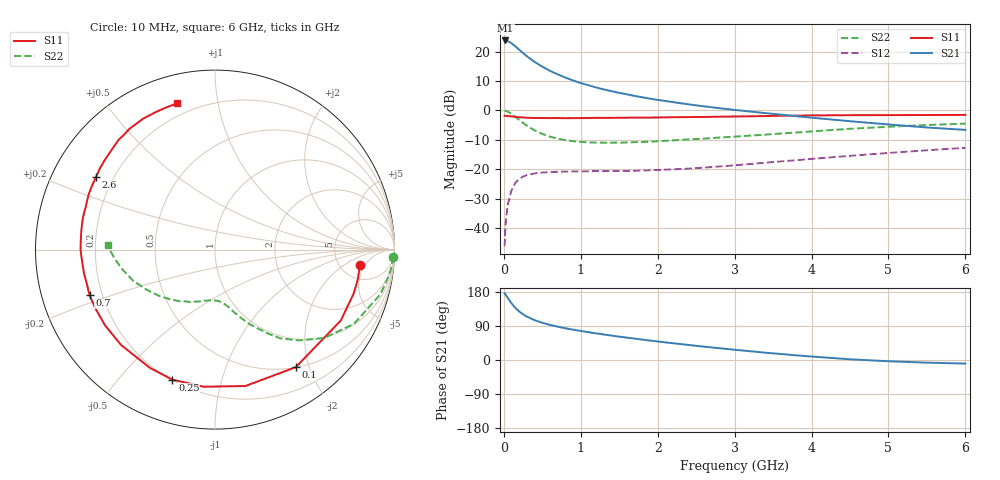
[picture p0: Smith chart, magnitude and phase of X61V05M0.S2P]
! SIEMENS Small Signal Semiconductors
! BFP193W
! Si NPN RF Bipolar Junction Transistor in SOT343
! VCE = 1 V  IC = 5 mA
! Common Emitter S-Parameters:  April 1994
# GHz  S  MA  R  50
!  f  S11  S21  S12  S22
! GHz  MAG  ANG  MAG  ANG  MAG  ANG  MAG  ANG
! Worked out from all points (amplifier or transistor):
!   40 points, 10 MHz to 6 GHz, reference 50 ohm
!   highest |S21| = 23.8 dB at 20 MHz (marker M1)
!   |S21| within 3 dB of that: start of sweep to 192.7 MHz
!   unconditionally stable (mu >= 1): 1.609 GHz to end of sweep
!   at 200 MHz: K = 0.15, MSG = 22.0 dB, |S12| = -23.3 dB
!   at 1.5 GHz: K = 0.95, MSG = 13.3 dB, |S12| = -20.6 dB
!   at 6 GHz: K = 1.01, MAG = 2.6 dB, |S12| = -12.7 dB
!   S11 on the Smith chart (normalised r, x): 10 MHz: 7.78, -3.83; 100 MHz: 0.50, -1.79; 250 MHz: 0.20, -0.71; 700 MHz: 0.15, -0.17; 2.6 GHz: 0.14, +0.28; 6 GHz: 0.14, +0.77
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0.01  0.8129 -5.9  15.56 176.0  0.0049 87.6  0.9929 -2.3
0.02  0.8127 -12.0  15.58 173.5  0.0101 83.0  0.9864 -6.3
0.03  0.8106 -17.6  15.51 170.3  0.0148 81.7  0.9766 -9.2
0.05  0.8048 -29.4  15.2 163.9  0.0244 75.2  0.9549 -15.1
0.1  0.7947 -55.5  13.93 149.5  0.0439 62.6  0.8782 -28.1
0.15  0.7787 -77.4  12.37 137.3  0.059 52.0  0.7826 -39.0
0.2  0.7666 -94.7  10.81 127.9  0.0682 44.4  0.6908 -47.1
0.25  0.7624 -108.1  9.517 120.5  0.0751 38.4  0.6162 -53.5
0.3  0.7522 -118.8  8.37 114.4  0.0796 34.0  0.5499 -58.0
0.4  0.7459 -134.6  6.723 105.1  0.0849 28.0  0.4591 -65.0
0.5  0.7438 -145.4  5.571 98.1  0.0878 24.3  0.4001 -69.8
0.6  0.7425 -153.6  4.73 92.5  0.0894 21.9  0.3591 -73.6
0.7  0.7437 -160.0  4.127 87.9  0.0906 20.4  0.3308 -76.4
0.9  0.7418 -169.7  3.249 80.0  0.0916 19.1  0.3 -81.7
1.1  0.745 -176.8  2.689 73.4  0.0924 18.8  0.286 -86.4
1.6  0.7541 169.2  1.883 58.9  0.0939 21.6  0.2856 -97.4
2.2  0.7684 156.4  1.387 44.2  0.0996 27.4  0.3098 -110.6
2.6  0.7765 148.5  1.178 35.2  0.1065 31.4  0.3316 -119.5
3.2  0.796 137.9  0.961 23.2  0.1226 35.7  0.3734 -132.2
4.5  0.8321 118.8  0.657 1.9  0.1691 37.2  0.4881 -159.2
5.5  0.8373 109.0  0.514 -7.0  0.2103 33.8  0.5659 -175.7
6  0.8415 104.5  0.468 -9.4  0.2316 31.6  0.5979 177.8
